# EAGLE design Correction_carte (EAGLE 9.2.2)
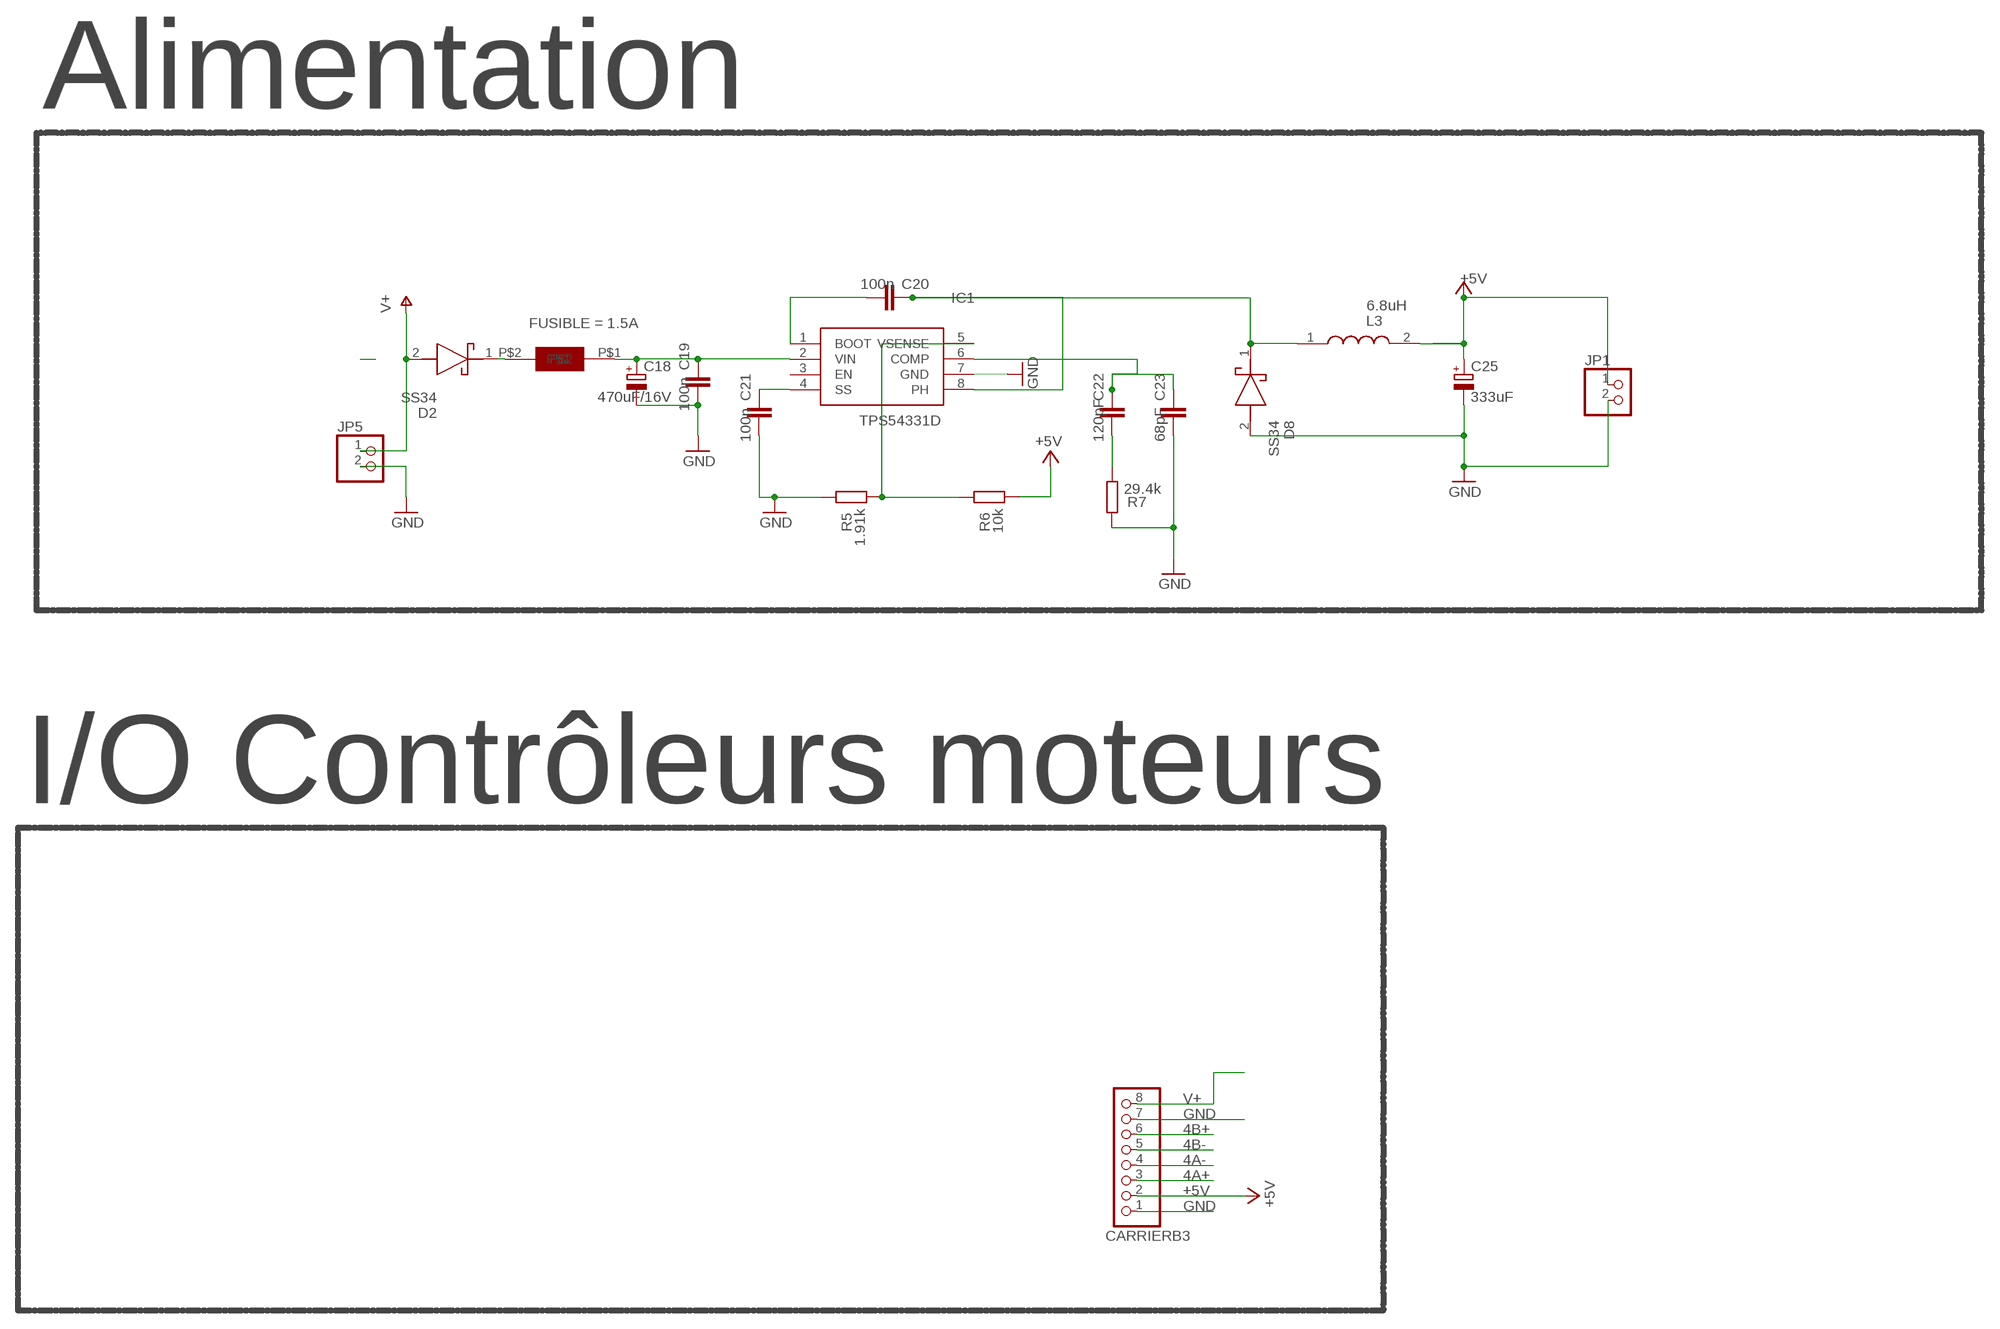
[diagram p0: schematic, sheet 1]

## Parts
C18  470uF/16V  CPOL-EUF  [PANASONIC_F]
C19  100n  C-EU0603-RND  [C0603-ROUND]
C20  100n  C-EU0603-RND  [C0603-ROUND]
C21  100n  C-EU0603-RND  [C0603-ROUND]
C22  120pF  C-EU0603-RND  [C0603-ROUND]
C23  68pF  C-EU0603-RND  [C0603-ROUND]
C25  333uF  CPOL-EUD  [PANASONIC_D]
CARRIERB3  PINHD-1X8  [1X08]
D2  SS34  [DIOM8059X256N]
D8  SS34  [DIOM8059X256N]
IC1  TPS54331D  [SOIC127P600X175-8N]
JP1  PINHD-1X2  [1X02]
JP5  PINHD-1X2  [1X02]
L3  6.8uH  7447709006  [WE-PD_1260/1245/1280/121054]
R5  1.91k  R-EU_R0603  [R0603-ROUND]
R6  10k  R-EU_R0603  [R0603-ROUND]
R7  29.4k  R-EU_R0603  [R0603-ROUND]
U$2  SMD-150  [SMDF-150]

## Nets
4A+: CARRIERB3.3
4A-: CARRIERB3.4
4B+: CARRIERB3.6
4B-: CARRIERB3.5
+5V: C25.+ CARRIERB3.2 JP1.1 L3.2 R6.1
GND: C18.- C19.1 C21.1 C23.1 C25.- CARRIERB3.1 CARRIERB3.7 D8.2(A) IC1.7(GND) JP1.2 JP5.2 R5.2 R7.2
N$2: C22.2 C23.2 IC1.6(COMP)
N$4: D2.1(K) U$2.P$2
N$5: C18.+ C19.2 IC1.2(VIN) U$2.P$1
N$6: C20.1 IC1.1(BOOT)
N$7: IC1.5(VSENSE) R5.1 R6.2
N$8: C21.2 IC1.4(SS)
N$9: C22.1 R7.1
N$13: C20.2 D8.1(K) IC1.8(PH) L3.1
V+: CARRIERB3.8 D2.2(A) JP5.1
Unconnected: IC1.3(EN)

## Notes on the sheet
- Alimentation
- I/O Contrôleurs moteurs

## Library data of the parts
C18 C25 = rcl:CPOL-EU: POLARIZED CAPACITOR, European symbol; SPICEPREFIX: C
C19-C23 = SmartPrj:C-EU: CAPACITOR, European symbol
CARRIERB3 = pinhead:PINHD-1X8: PIN HEADER
D2 D8 = SamacSys_Parts:SS34: ON Semi SS34 SMT Schottky Diode, 40V 3A, 2-Pin DO-214AB; DESCRIPTION: ON Semi SS34 SMT Schottky Diode, 40V 3A, 2-Pin DO-214AB; HEIGHT: 2.56mm; MANUFACTURER_NAME: ON Semiconductor; MANUFACTURER_PART_NUMBER: SS34; RS_PART_NUMBER: 1662321
IC1 = SamacSys_Parts:TPS54331D: Texas Instruments, TPS54331D Step-Down Switching Regulator 3A Adjustable, Minimum of 0.8 V, 8-Pin SOIC Source: Datasheet; DESCRIPTION: Texas Instruments, TPS54331D Step-Down Switching Regulator 3A Adjustable, Minimum of 0.8 V, 8-Pin SOIC; HEIGHT: mm; MANUFACTURER_NAME: Texas Instruments; MANUFACTURER_PART_NUMBER: TPS54331D; RS_PART_NUMBER: 6618521P; RS_PRICE-STOCK: http://uk.rs-online.com/web/p/products/6618521P
JP1 JP5 = pinhead:PINHD-1X2: PIN HEADER
L3 = SamacSys_Parts:7447709006: Wurth WE-PD Series Shielded Wire-wound SMD Inductor 6.8 uH +/-20% 8.4A Idc; DESCRIPTION: Wurth WE-PD Series Shielded Wire-wound SMD Inductor 6.8 uH +/-20% 8.4A Idc; HEIGHT: mm; MANUFACTURER_NAME: Wurth Elektronik; MANUFACTURER_PART_NUMBER: 7447709006; RS_PART_NUMBER: 7896776; RS_PRICE-STOCK: http://uk.rs-online.com/web/p/products/7896776
R5-R7 = SmartPrj:R-EU_: RESISTOR, European symbol
U$2 = MyLib:SMD-150; FUSIBLE: 1.5A

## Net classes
0 default: width 0.15 mm, drill 0.3 mm, clearance 0.15 mm

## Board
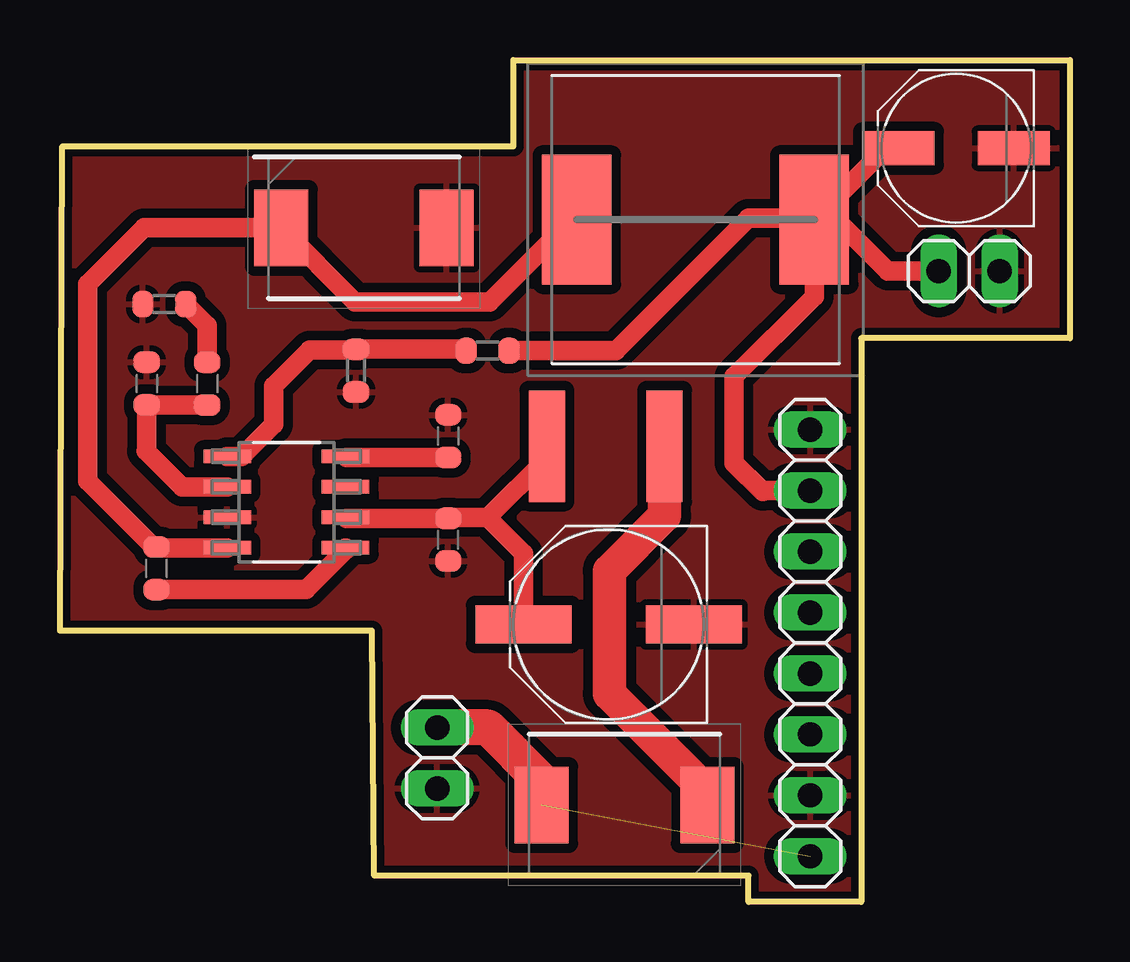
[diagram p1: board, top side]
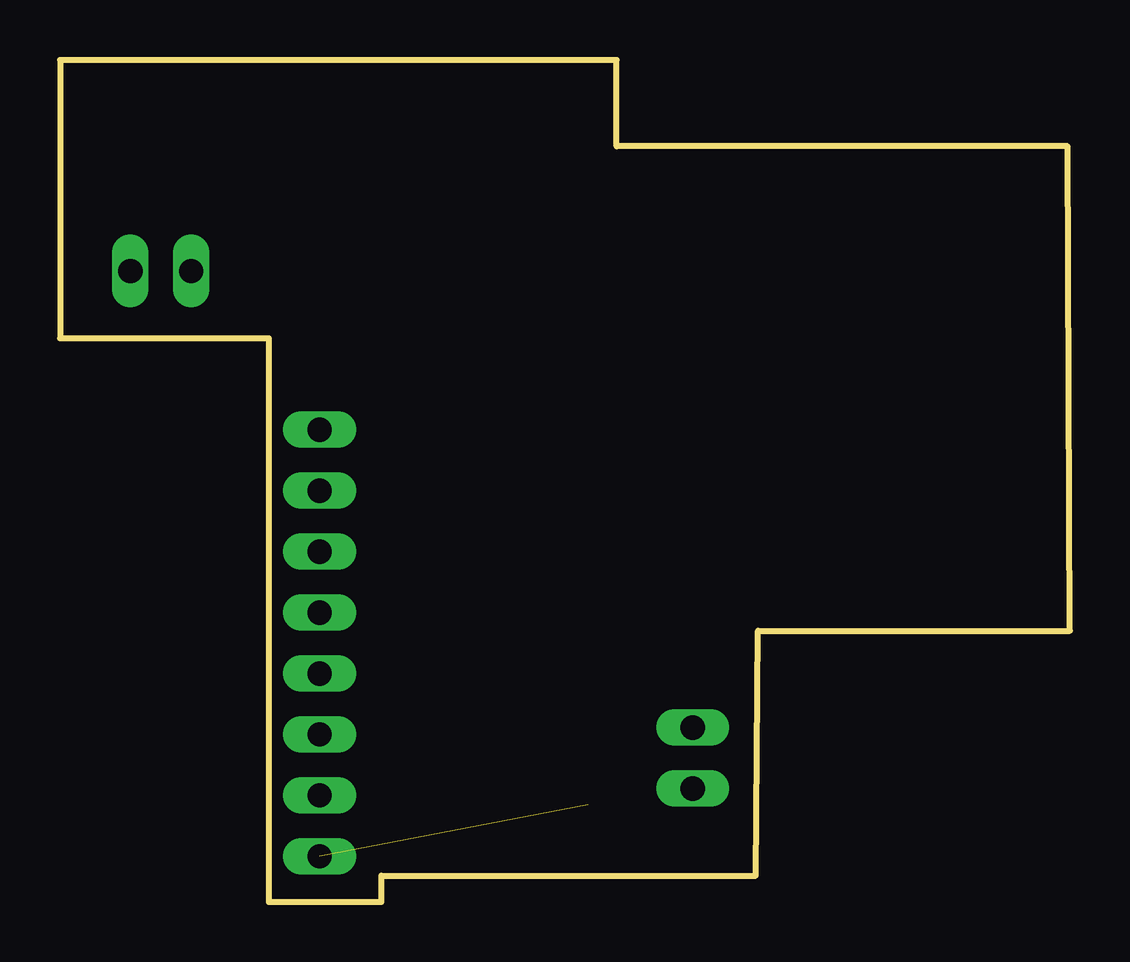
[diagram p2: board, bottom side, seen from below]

Size 42.1 x 35.1 mm. Coordinates in mm from the lower left corner, seen from the top.
Outline: 33.4,0 28.7,0 28.7,1.1 13.1,1.1 13,11.3 0,11.3 0.1,31.5 18.9,31.5 18.9,35.1 42.1,35.1 42.1,23.5 33.4,23.5 33.4,0
Copper layers (1*16): Top 0.035mm / dielectric 1.5mm / Bottom 0.035mm
Design rules "default *": minimum track width 0.15mm, minimum drill 0.3mm, track to track 0.4mm, track to pad 0.4mm, pad to pad 0.4mm, via to via 0.15mm, smd to smd 0.15mm, copper to edge 0.3mm, drill to drill 0.3mm, minimum pad ring 10mil, minimum via ring 10mil, stop-mask expansion 2mil, vias tented up to drill 1mil, thermal gap 10mil

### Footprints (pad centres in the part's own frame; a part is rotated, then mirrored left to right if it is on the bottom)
PANASONIC_F = smd 4 x 1.6: + 3.55,0; - -3.55,0
C0603-ROUND = smd 0.898 x 1.1: 1 -0.889,0; 2 0.889,0
PANASONIC_D = smd 3 x 1.4: + 2.4,0; - -2.4,0
1X08 = drill 1.016 long: 1 -8.89,0; 2 -6.35,0; 3 -3.81,0; 4 -1.27,0; 5 1.27,0; 6 3.81,0; 7 6.35,0; 8 8.89,0
DIOM8059X256N = smd 2.25 x 3.2: 1 -3.45,0; 2 3.45,0
SOIC127P600X175-8N = smd 1.981 x 0.559: 1 -2.464,1.905; 2 -2.464,0.635; 3 -2.464,-0.635; 4 -2.464,-1.905; 5 2.464,-1.905; 6 2.464,-0.635; 7 2.464,0.635; 8 2.464,1.905
1X02 = drill 1.016 long: 1 -1.27,0; 2 1.27,0
WE-PD_1260/1245/1280/121054 = smd 2.9 x 5.4: 1 -4.95,0; 2 4.95,0
R0603-ROUND = smd 0.898 x 1.1: 1 -0.889,0; 2 0.889,0
SMDF-150 = smd 1.5 x 4.65: P$1 -2.4,0; P$2 2.5,0

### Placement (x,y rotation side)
C18  22.87,11.57 180 top
C19  16.18,15.1 90 top
C20  4.02,13.91 90 top
C21  16.18,19.42 270 top
C22  6.13,21.61 270 top
C23  3.61,21.61 270 top
C25  37.35,31.43 180 top
CARRIERB3  31.28,10.79 270 top
D2  23.53,4.04 180 top
D8  12.67,28.1 0 top
IC1  9.44,16.67 180 top
JP1  37.9,26.3 0 top
JP5  15.73,6 270 top
L3  26.5,28.45 0 top
R5  12.34,22.15 270 top
R6  17.83,22.98 180 top
R7  4.35,24.92 180 top
U$2  22.7,19 0 top

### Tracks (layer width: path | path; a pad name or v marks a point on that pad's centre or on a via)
+5V
  Top 0.61: 29.3,17.1 29.34,17.14 | 31.39,28.5 L3.2
  Top 0.813: C25.+ 34.43,31.43 L3.2 | L3.2 31.44,25.25 28.1,21.9 28.1,18.3 29.3,17.1 | 29.34,17.14 CARRIERB3.2 | R6.1 23.18,22.98 28.7,28.5 31.39,28.5 | L3.2 32.45,28.45 | L3.2 32.36,28.45 34.5,26.3 JP1.1
  Top 1.016: 30.65,28.45 L3.2
GND
  pour Top: 0.1,31.5 0.1,11.3 13.1,11.3 13.1,1 28.7,1.1 28.7,0.1 33.4,0.1 33.4,23.5 42.1,23.5 42.1,35.1 18.9,35.1 18.9,31.5
N$2
  Top 0.61: C22.2 | 3.6,18.8 3.61,18.81
  Top 0.813: C22.2 C23.2 3.61,18.81 | IC1.6 5.09,17.31 3.6,18.8
N$4
  Top 1.4: U$2.P$2 25.2,16.1 22.9,13.8 22.9,8.68 26.98,4.6 D2.1
N$5
  Top 0.508: C19.2 16.21,16.02 | 11.95,15.99 IC1.2
  Top 0.813: 17.83,16.02 19.32,14.53 C18.+ | 17.83,16.02 16.21,16.02 | C19.2 11.95,15.99 | 17.83,16.02 20.3,18.49
  Top 1.27: 20.3,18.49 U$2.P$1
N$6
  Top 0.813: C20.1 4.03,13.03 10.27,13.03 11.9,14.67 IC1.1
N$7
  Top 0.61: 12.31,23 R5.1 | 16.88,23.04 R6.2
  Top 0.813: IC1.5 7.58,18.58 8.9,19.9 8.9,21.5 10.4,23 12.31,23 | R5.1 16.88,23.04
N$8
  Top 0.508: 11.95,18.53 IC1.4
  Top 0.813: C21.2 11.95,18.53
N$9
  Top 0.813: R7.1 6.13,24.02 C22.1
N$13
  Top 0.61: 4.05,14.77 C20.2
  Top 0.813: L3.1 21.34,28.45 17.91,25.02 12.31,25.02 D8.1 3.5,28.1 1.16,25.75 1.16,17.54 3.9,14.8 C20.2 | IC1.8 4.05,14.77
V+  (1 unrouted)
  Top 1.5: D2.2 20.08,5.04 17.85,7.27 JP5.1
  Bottom 1.5: JP5.1 15.73,7.29

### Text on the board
ReferenceLC: L | TX | RX | PC1 | PC2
